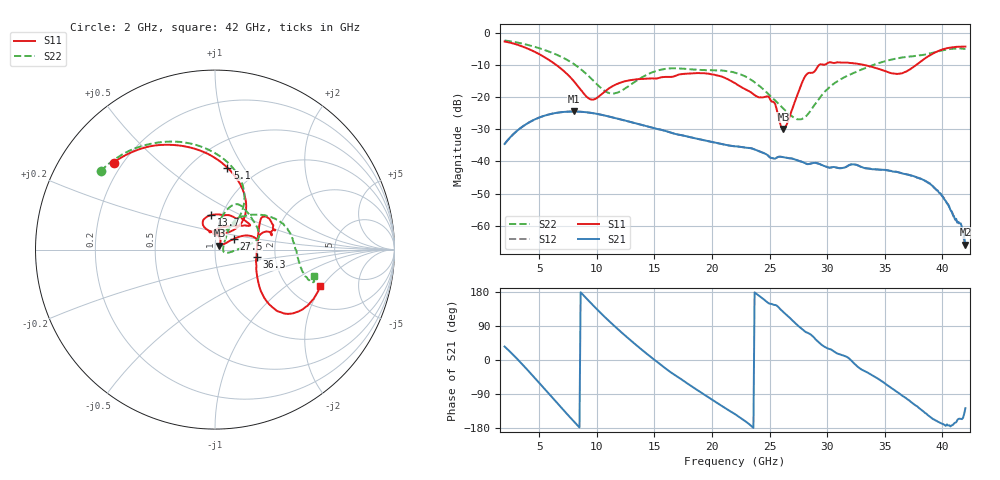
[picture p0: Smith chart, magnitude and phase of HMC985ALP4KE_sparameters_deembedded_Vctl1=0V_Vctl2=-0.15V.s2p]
!s2p File: Measurements: S11, S21, S12, S22
# GHz S dB R 50.0
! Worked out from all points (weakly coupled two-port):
!   401 points, 2 GHz to 42 GHz, reference 50 ohm
!   highest |S21| = -24.41 dB at 8 GHz (marker M1); lowest = -65.9 dB at 42 GHz (marker M2)
!   lowest |S11| = -29.8 dB at 26.2 GHz (marker M3), VSWR 1.07, Z = 52.5 + j2.21 ohm
!   |S11| at or under -10 dB: 6.528 GHz to 29.27 GHz (22.75 GHz wide, 127 % of centre); 33.34 GHz to 37.69 GHz (4.352 GHz wide, 12.3 % of centre)
!   |S22| runs from -26.9 to -2.2 dB; largest |S21 - S12| = 0.00013
!   S11 on the Smith chart (normalised r, x): 2 GHz: 0.17, +0.36; 5.1 GHz: 0.73, +0.85; 13.7 GHz: 0.89, +0.35; 27.5 GHz: 1.22, +0.15; 36.3 GHz: 1.59, -0.14; 42 GHz: 2.90, -1.91
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2  -2.56 139.4  -34.54 35.5  -34.54 35.4  -2.24 145.5
3.5  -4.07 111.4  -29.26 -10.3  -29.27 -10.3  -3.20 121.8
5.1  -6.71 81.5  -26.16 -63.6  -26.17 -63.6  -4.77 97.4
8  -14.89 44.8  -24.41 -161.8  -24.41 -161.8  -9.56 60.4
8.7  -18.06 51.5  -24.51 175.4  -24.52 175.4  -11.46 55.3
9.7  -20.68 87.2  -24.94 143.6  -24.95 143.6  -14.80 53.2
11.2  -16.88 115.8  -26.09 98.9  -26.09 98.9  -18.75 68.2
13.7  -14.29 96.7  -28.39 32.4  -28.40 32.4  -14.23 77.3
15.4  -13.94 73.0  -29.96 -8.5  -29.96 -8.5  -11.51 68.3
19.4  -12.51 34.7  -33.47 -92.7  -33.47 -92.7  -11.50 34.4
22  -15.56 52.2  -35.26 -142.9  -35.27 -143.0  -12.28 13.5
25  -20.23 97.6  -38.64 148.6  -38.63 148.6  -19.31 -3.4
26.2  -29.83 40.7  -38.67 126.3  -38.67 126.3  -23.51 -15.5
27.5  -18.43 29.5  -39.77 89.7  -39.73 89.6  -26.83 -3.1
28.1  -13.37 20.6  -40.54 74.8  -40.59 74.7  -26.12 19.9
28.7  -12.32 12.8  -40.56 64.0  -40.53 64.0  -23.42 38.3
31  -9.10 23.3  -42.05 15.9  -42.09 16.1  -14.70 56.5
35.4  -12.27 12.4  -42.92 -70.0  -42.88 -70.1  -8.37 26.0
36.3  -12.57 -10.1  -43.50 -89.4  -43.49 -89.5  -7.69 18.1
39.6  -5.63 -42.8  -49.07 -162.7  -49.23 -161.4  -5.71 -15.8
41.5  -4.18 -23.1  -59.30 -154.9  -59.69 -155.6  -4.72 -17.6
42  -4.14 -19.1  -65.91 -127.1  -66.43 -130.1  -4.88 -14.7
